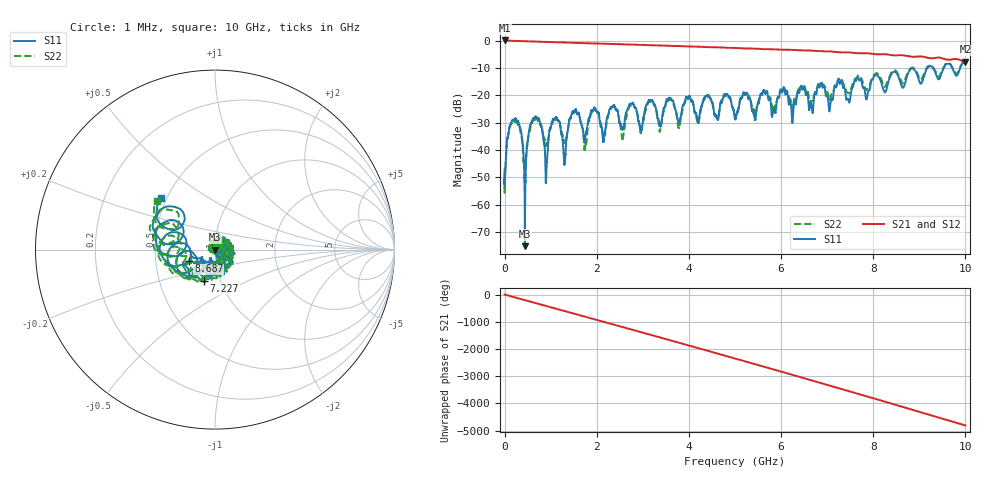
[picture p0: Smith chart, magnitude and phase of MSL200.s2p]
! 3/21/2017 9:37:04 AM
! F:\HUSERTL_20170321\MSL200.S2P
! CHANNEL.1
! TR.MEASUREMENT
! CORRECTED.DATA
# GHZ S RI R 50.0
! FREQ.GHZ  S11RE  S11IM  S31RE  S31IM  S13RE  S13IM  S33RE  S33IM
!; PortSelection: Port_13
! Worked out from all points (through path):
!   10000 points, 1 MHz to 10 GHz, reference 50 ohm
!   highest |S21| = 0.04 dB at 10 MHz (marker M1); lowest = -7.8 dB at 10 GHz (marker M2)
!   group delay of S21, straight-line fit = 1.33 ns
!   lowest |S11| = -75.2 dB at 441 MHz (marker M3), VSWR 1.00, Z = 50 - j0.0167 ohm
!   |S11| at or under -10 dB: start of sweep to 9.175 GHz; 9.294 GHz to 9.532 GHz (237.8 MHz wide, 2.53 % of centre); 9.713 GHz to 9.888 GHz (175 MHz wide, 1.79 % of centre)
!   |S22| runs from -55.7 to -7.5 dB; largest |S21 - S12| = 0.045
!   S11 on the Smith chart (normalised r, x): 1 MHz: 1.01, +0.00; 7.227 GHz: 0.84, -0.30; 8.687 GHz: 0.74, -0.10; 10 GHz: 0.47, +0.33
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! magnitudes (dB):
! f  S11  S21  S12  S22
! 1 MHz  -50.8  0.0  0.0  -53.6
! 10 MHz  -50.4  0.0  0.0  -48.8
! 212 MHz  -28.9  -0.1  -0.2  -29.3
! 441 MHz  -75.2  -0.2  -0.3  -51.0
! 647 MHz  -28.4  -0.4  -0.4  -29.0
! 897 MHz  -50.9  -0.5  -0.5  -38.1
! 1.079 GHz  -28.8  -0.6  -0.6  -29.3
! 1.297 GHz  -44.5  -0.7  -0.7  -37.2
! 1.483 GHz  -25.8  -0.8  -0.8  -26.4
! 1.668 GHz  -30.8  -0.9  -0.9  -30.7
! 3.164 GHz  -21.9  -1.7  -1.7  -22.5
! 3.334 GHz  -28.8  -1.8  -1.8  -28.9
! 3.981 GHz  -21.0  -2.1  -2.2  -21.2
! 5.001 GHz  -28.6  -2.7  -2.7  -27.3
! 5.22 GHz  -19.9  -2.9  -2.9  -19.4
! 5.416 GHz  -27.4  -3.0  -3.0  -25.6
! 5.649 GHz  -19.1  -3.2  -3.2  -18.7
! 6.667 GHz  -24.4  -3.7  -3.8  -22.1
! 7.227 GHz  -14.7  -4.2  -4.3  -14.9
! 8.334 GHz  -14.7  -5.1  -5.2  -14.0
! 8.687 GHz  -15.9  -5.5  -5.5  -14.4
! 10 GHz  -7.6  -7.8  -7.8  -7.5
